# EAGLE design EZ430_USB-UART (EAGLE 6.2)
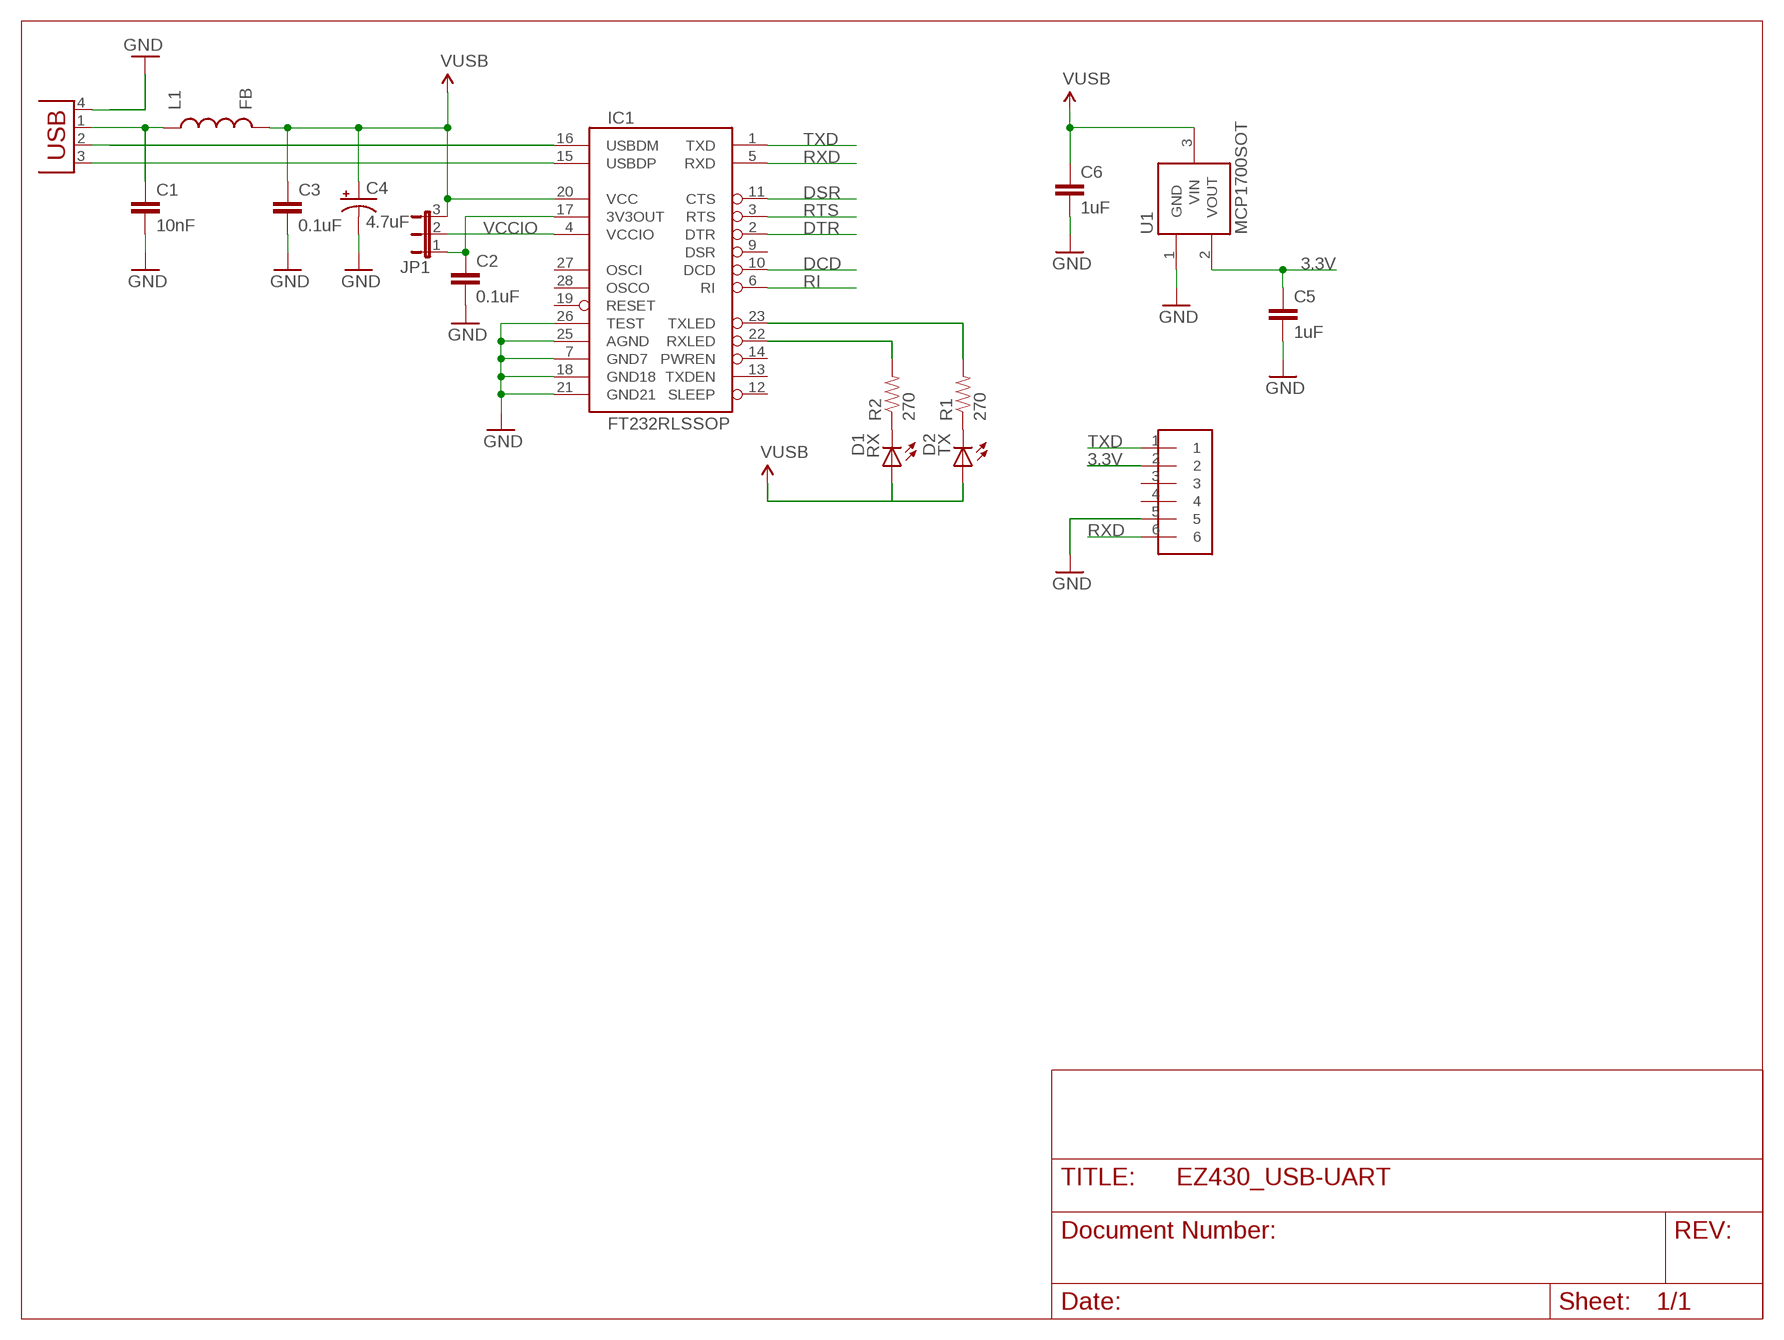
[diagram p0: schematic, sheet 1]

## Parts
C1  10nF  CAP0603  [0603]
C2  0.1uF  CAP0603  [0603]
C3  0.1uF  CAP0603  [0603]
C4  4.7uF  CAP_POL1206  [EIA3216]
C5  1uF  CAP0805  [0805]
C6  1uF  CAP0805  [0805]
H1  HEADER-6MILL-MAX  [MILL-MAX-6PIN-EZ430-RF2500]
IC1  FT232RLSSOP  [SSOP28DB]
JP1  JUMPER-3PTH  [1X03]
L1  FB  INDUCTOR0603  [0603]
R1  270  RESISTOR  [0805]
R2  270  RESISTOR  [0805]
RX  D1  LED0603  [LED-0603]
TX  D2  LED0603  [LED-0603]
U1  MCP1700SOT  [SOT23-3]
X1  USB  [KUSBX-SMT2AP1S-B]

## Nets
3.3V: C5.1 H1.2 U1.2(VOUT)
D+: IC1.15(USBDP) X1.3(D+)
D-: IC1.16(USBDM) X1.2(D-)
DCD: IC1.10(DCD)
DSR: IC1.11(CTS)
DTR: IC1.2(DTR)
GND: C1.2 C2.2 C3.2 C4.C(-) C5.2 C6.2 H1.5 IC1.7(GND7) IC1.18(GND18) IC1.21(GND21) IC1.25(AGND) IC1.26(TEST) U1.1(GND) X1.4(GND)
N$1: IC1.22(RXLED) R2.2
N$2: IC1.23(TXLED) R1.2
N$3: C2.1 IC1.17(3V3OUT) JP1.1
N$4: R2.1 RX.C
N$5: R1.1 TX.C
RI: IC1.6(RI)
RTS: IC1.3(RTS)
RXD: H1.6 IC1.5(RXD)
TXD: H1.1 IC1.1(TXD)
VCC: C3.1 C4.A(+) C6.1 IC1.20(VCC) JP1.3 L1.2 RX.A TX.A U1.3(VIN) ; supply symbol labelled VUSB
VCCIO: IC1.4(VCCIO) JP1.2
VUSB: C1.1 L1.1 X1.1(VBUS)
Unconnected: H1.3 H1.4 IC1.9(DSR) IC1.12(SLEEP) IC1.13(TXDEN) IC1.14(PWREN) IC1.19(RESET) IC1.27(OSCI) IC1.28(OSCO)

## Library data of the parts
C1-C3 C5 C6 = SparkFun:CAP: Capacitor
C4 = SparkFun:CAP_POL: Capacitor Polarized
H1 = gustavo:HEADER-6
IC1 = SparkFun:FT232RL: USB UART FT232RL 4th Generation USB UART (USB <-> Serial) Controller. Spark Fun Electronics SKU : COM-00650
JP1 = SparkFun:JUMPER-3
L1 = gustavo:INDUCTOR: Inductors
R1 R2 = SparkFun:RESISTOR: Resistor
RX TX = SparkFun:LED: LEDs
U1 = gustavo:MCP1700; DIGIKEY#: 321432
X1 = gustavo:USB: USB Connectors USB-B-PTH is fully proven SKU : PRT-00139 USB-miniB is fully proven SKU : PRT-00587 USB-A-PCB is untested. USB-A-H is throughly reviewed, but untested. Spark Fun Electronics SKU : PRT-00437 USB-B-SMT is throughly reviewed, but untested. Needs silkscreen touching up. USB-A-S has not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

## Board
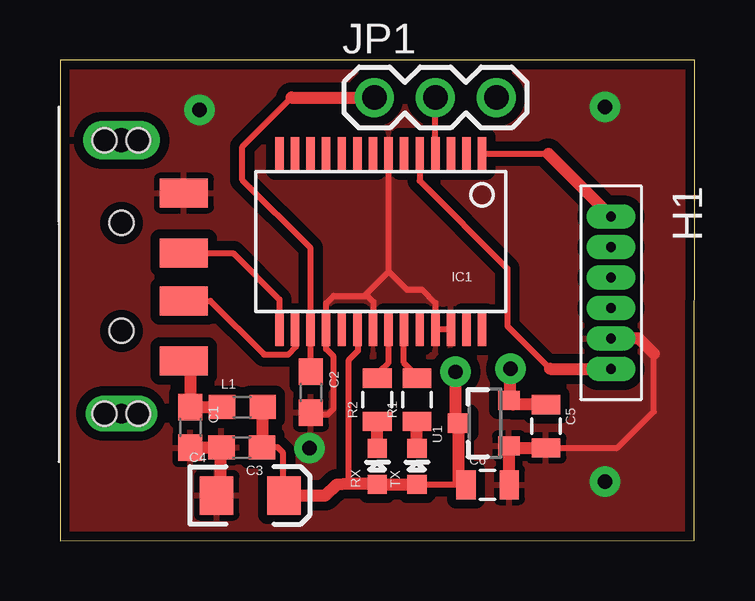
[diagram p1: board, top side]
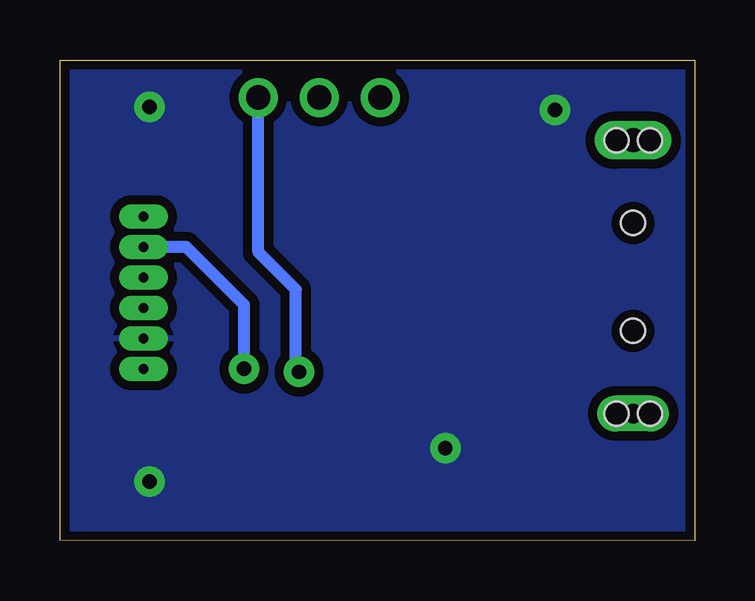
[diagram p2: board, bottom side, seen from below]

Size 26.44 x 20.04 mm. Coordinates in mm from the lower left corner, seen from the top.
Outline: 0,0 26.43,0.01 26.44,20.04 0,20.04 0,0
Copper layers (1*16): Top 0.0356mm / dielectric 1.5011mm / Bottom 0.0356mm
Design rules: minimum track width 8mil, minimum drill 20mil, track to track 8mil, track to pad 8mil, pad to pad 8mil, via to via 8mil, smd to smd 8mil, copper to edge 10mil, drill to drill 8mil, minimum pad ring 12mil, minimum via ring 10mil, stop-mask expansion 4mil, vias tented up to drill 25mil, thermal gap 10mil

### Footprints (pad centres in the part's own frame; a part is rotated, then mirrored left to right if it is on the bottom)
0603 = smd 1.1 x 1: 1 -0.85,0; 2 0.85,0
EIA3216 = smd 1.4 x 1.6: A 1.4,0; C -1.4,0
0805 = smd 0.8 x 1.2: 1 -0.9,0; 2 0.9,0
MILL-MAX-6PIN-EZ430-RF2500 = drill 0.406 long: 1 -2.54,0; 2 -1.27,0; 3 0,0; 4 1.27,0; 5 2.54,0; 6 3.81,0
SSOP28DB = smd 0.348 x 1.397: 1 -4.225,-3.656; 2 -3.575,-3.656; 3 -2.925,-3.656; 4 -2.275,-3.656; 5 -1.625,-3.656; 6 -0.975,-3.656; 7 -0.325,-3.656; 8 0.325,-3.656; 9 0.975,-3.656; 10 1.625,-3.656; 11 2.275,-3.656; 12 2.925,-3.656; 13 3.575,-3.656; 14 4.225,-3.656; 15 4.225,3.656; 16 3.575,3.656; 17 2.925,3.656; 18 2.275,3.656; 19 1.625,3.656; 20 0.975,3.656; 21 0.325,3.656; 22 -0.325,3.656; 23 -0.975,3.656; 24 -1.625,3.656; 25 -2.275,3.656; 26 -2.925,3.656; 27 -3.575,3.656; 28 -4.225,3.656
1X03 = drill 1.016: 1 0,0; 2 2.54,0; 3 5.08,0
LED-0603 = smd 0.8 x 0.8: A 0,-0.75; C 0,0.75
SOT23-3 = smd 0.8 x 0.9: 1 -0.95,-1; 2 0.95,-1; 3 0,1.1
KUSBX-SMT2AP1S-B = smd 1.2 x 2: 1 -3.5,4; 2 -6,4; 3 -8,4; 4 -10.5,4 | drill 1 pad 1.5 long: P$5 -12.7,1.4 | drill 0.8 pad 1.5 long: P$6 -1.3,1.4 | hole 1: -4.75,1.4; -9.25,1.4; -12.7,2.1; -12.7,0.7; -1.3,2.1; -1.3,0.7

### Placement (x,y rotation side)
C1  5.43,4.72 270 top
C2  10.45,6.19 270 top
C3  7.57,3.89 180 top
C4  7.93,1.88 0 top
C5  20.25,4.77 270 top
C6  17.82,2.33 0 top
H1  22.96,10.97 270 top
IC1  13.36,12.47 180 top
JP1  13.1,18.47 0 top
L1  7.6,5.57 0 top
R1  14.87,5.87 90 top
R2  13.22,5.87 90 top
RX  13.22,3.1 0 top
TX  14.87,3.1 0 top
U1  17.71,4.9 90 top
X1  1.16,4 270 top

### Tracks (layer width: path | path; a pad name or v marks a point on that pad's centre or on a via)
3.3V  (via drill 0.6 pad 1.27)
  Top 0.254: 18.88,5.67 U1.2 18.77,5.78
  Top 0.508: C5.1 18.88,5.67 | 18.77,5.78 v18.77,7.16
  Bottom 0.508: H1.2 21.18,12.24 18.77,9.83 v18.77,7.16
D+
  Top 0.254: IC1.15 9.14,10.06 7.21,11.99 5.17,11.99 X1.3
D-
  Top 0.254: IC1.16 9.83,8.73 9.83,8.09 9.5,7.76 8.5,7.76 6.27,10 X1.2
GND  (via drill 0.6 pad 1.27)
  Top 0.254: 18.76,3.87 U1.1 18.72,3.81 | C6.2 18.75,2.17 | 6.7,3.87 C3.2 | C4.C 6.7,2.06 | 12.67,10.21 12.8,10.21 13.06,9.96 13.06,8.83 IC1.21 | 12.67,10.21 11.4,10.21 11.09,9.89 IC1.18 11.09,7.99 11.4,7.67 11.4,5.51 11.15,5.26 10.53,5.26 C2.2 | 13.69,11.22 IC1.7 | 12.67,10.21 13.69,11.22 | C5.2 23.23,3.87 24.74,5.38 24.74,7.8 | IC1.26 IC1.25 15.64,9.91 15.09,10.46 14.45,10.46 13.69,11.22
  Top 0.508: 18.76,3.87 C5.2 | C6.2 18.72,3.81 | C1.2 6.7,3.87 6.7,2.06 | 24.74,7.8 24.1,8.43 H1.5
  other vias: 10.39,3.86 5.82,17.96 22.71,18.08 22.71,2.46
  pour Top (isolate 0.381): 0.1,20.12 0.1,-0.08 26.26,-0.08 26.39,0.05 26.39,19.86 26.26,19.99
  pour Bottom (isolate 0.381): 0.36,19.74 0.36,0.56 0.23,0.43 25.88,0.43 26.01,0.56 26.01,19.61 25.88,19.74
N$1
  Top 0.254: R2.2 13.35,7.07 13.69,7.42 IC1.22
N$2
  Top 0.254: R1.2 15,6.74 14.33,7.42 14.33,8.8 IC1.23
N$3
  Top 0.254: C2.1 10.44,7.05 IC1.17 10.44,12.19 7.59,15.04 7.59,16.43 9.64,18.47
  Top 0.508: 9.64,18.47 JP1.1
N$4
  Top 0.508: RX.C R2.1
N$5
  Top 0.508: TX.C R1.1
N$6  (via drill 0.6 pad 1.27)
  other vias: 18.77,7.16
RXD
  Top 0.254: IC1.5 14.99,15.01 18.64,11.35 18.64,8.94 20.42,7.16
  Top 0.508: 20.42,7.16 H1.6
TXD
  Top 0.254: IC1.1 20.34,16.13
  Top 0.508: 20.34,16.13 H1.1
VCC  (via drill 0.6 pad 1.27)
  Top 0.254: C3.1 8.45,3.92 | C3.1 9.06,3.89 9.3,3.65 9.3,1.91 C4.A | C3.1 8.65,4.11 | TX.A 16.77,2.35 C6.1 16.61,2.51 | 13.17,2.39 RX.A | U1.3 16.48,4.89 | IC1.20 12.42,8.79 12.42,7.92 12.04,7.54 12.04,2.39
  Top 0.508: 8.45,3.92 L1.2 | RX.A TX.A | 16.61,2.51 U1.3 | C4.A 11.05,1.88 11.53,2.34 12.04,2.39 13.17,2.39 | 16.48,4.89 v16.48,7.04
  Bottom 0.254: v16.48,7.04 16.61,7.16
  Bottom 0.508: JP1.3 18.18,12.03 16.61,10.46 16.61,7.16
VCCIO
  Top 0.254: IC1.4 JP1.2
VUSB
  Top 0.254: L1.1 | X1.1 5.43,7.23
  Top 0.508: L1.1 C1.1 5.43,7.23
